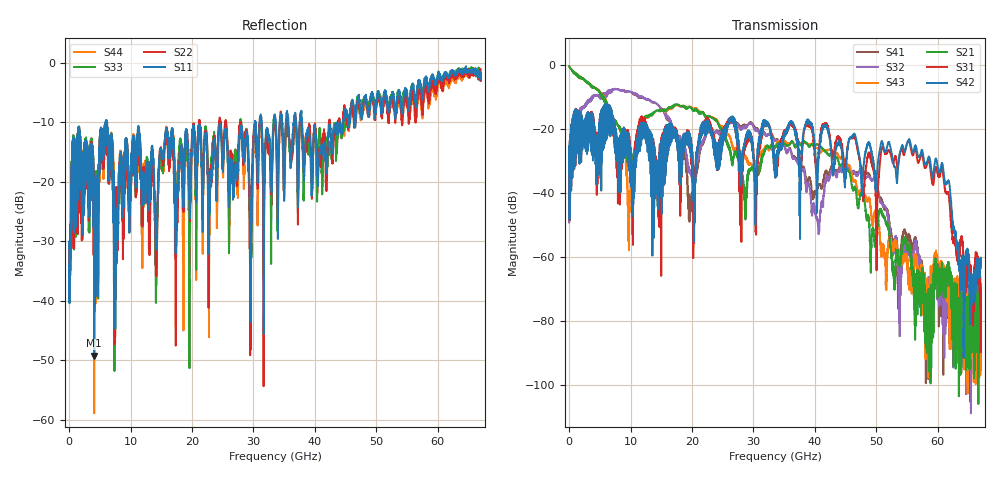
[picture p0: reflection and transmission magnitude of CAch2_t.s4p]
!Agilent Technologies,N5247A,US51170199,A.09.90.13
!Agilent N5247A: A.09.90.13
!Date: Wednesday, October 17, 2018 15:31:34
!Correction: S11(Full 4 Port(1,2,3,4))
!S12(Full 4 Port(1,2,3,4))
!S13(Full 4 Port(1,2,3,4))
!S14(Full 4 Port(1,2,3,4))
!S21(Full 4 Port(1,2,3,4))
!S22(Full 4 Port(1,2,3,4))
!S23(Full 4 Port(1,2,3,4))
!S24(Full 4 Port(1,2,3,4))
!S31(Full 4 Port(1,2,3,4))
!S32(Full 4 Port(1,2,3,4))
!S33(Full 4 Port(1,2,3,4))
!S34(Full 4 Port(1,2,3,4))
!S41(Full 4 Port(1,2,3,4))
!S42(Full 4 Port(1,2,3,4))
!S43(Full 4 Port(1,2,3,4))
!S44(Full 4 Port(1,2,3,4))
!S4P File: Measurements: <S11,S12,S13,S14>,
!<S21,S22,S23,S24>,
!<S31,S32,S33,S34>,
!<S41,S42,S43,S44>:
# Hz S  dB  R 50
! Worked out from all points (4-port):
!   6701 points, 10 MHz to 67 GHz, reference 50 ohm
!   strongest paths, dB at 10 MHz, 16.76 GHz, 33.51 GHz, 50.25 GHz, 67 GHz:
!     S42: -33.4, -22.9, -29.3, -30.3, -60.6
!     S31: -33.4, -22.2, -28.5, -37.8, -76.5
!     S21: -0.3, -12.8, -25.4, -49.1, -71.3
!     S43: -0.3, -13.0, -25.8, -46.9, -77.6
!     S32: -49.1, -18.8, -23.7, -38.3, -81.3
!     S41: -49.0, -19.2, -23.3, -39.2, -77.3
!   lowest |S11| = -49.2 dB at 4.089 GHz (marker M1), VSWR 1.01, Z = 49.7 + j0.0126 ohm
!   |S11| at or under -10 dB: start of sweep to 5.967 GHz; 6.191 GHz to 30.23 GHz (24.03 GHz wide, 132 % of centre); 37.92 GHz to 44.09 GHz (6.175 GHz wide, 15.1 % of centre)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
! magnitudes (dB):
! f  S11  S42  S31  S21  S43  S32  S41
! 10 MHz  -31.0  -33.4  -33.4  -0.3  -0.3  -49.1  -49.0
! 4.089 GHz  -49.2  -27.1  -24.9  -6.9  -6.8  -9.4  -9.3
! 9.749 GHz  -21.0  -31.4  -25.6  -31.4  -57.8  -8.1  -8.2
! 19.62 GHz  -22.6  -24.9  -25.5  -13.0  -12.8  -32.7  -45.6
! 29.58 GHz  -41.3  -21.9  -21.8  -32.7  -30.8  -18.2  -17.9
! 55.21 GHz  -7.0  -23.4  -23.5  -56.9  -64.4  -56.8  -54.0
! 67 GHz  -2.6  -60.6  -76.5  -71.3  -77.6  -81.3  -77.3
